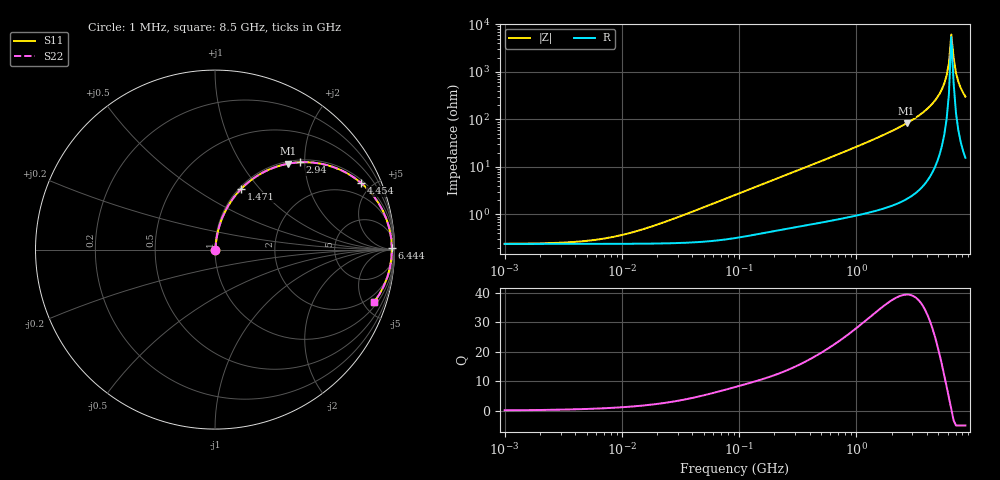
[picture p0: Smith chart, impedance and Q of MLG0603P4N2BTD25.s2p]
! S-Parameter Data Generated by TDK Corporation
! Copyright(C) 2025 TDK Corporation.
! All Rights Reserved.
! TDK P/N: MLG0603P4N2BTD25 (SMD / SMT Inductor (Coil))
! Property: L=4.2nH at 500MHz
! Size(LxWxT): 0.6x0.3x0.3mm
! Model Type: s2p (Touchstone File Format Version 1.0)
! Frequency: DC=Yes Start=1MHz Stop=8500MHz 198points Log-sweep
! Model Generated on Feb. 6, 2025
! Terms and conditions regarding TDK Simulation Models:
! 1)This simulation model is being provided solely for informational
!  purposes. Please refer to the specifications of the products in
!  terms of detailed characteristics of such products.
! 2)In no event shall TDK Corporation of any of its subsidiaries be
!  liable for any loss or damage arising, directly or indirectly,
!  from any information contained in this simulation model, including,
!  but not limited to loss or damages arising from any inaccuracies,
!  omissions or errors in connection with such information.
! 3)Any and all copyrights on this simulation model are owned by
!  TDK Corporation.  Duplication or redistribution of this simulation
!  model without prior written permission from TDK Corporation
!  is prohibited.
! 4)This simulation model is subject to any modification or change
!  without any prior notice.
! 5)Neither TDK Corporation nor any of its subsidiaries shall make any
!  warranty, express or implied, including but not limited to the
!  correctness, implied warranties of merchantability and fitness for
!  a particular purpose with respect to this simulation models.
! 6)The use of this simulation model shall be deemed to have consented
!  to the terms and conditions hereof.
! Port Assignments:
!  1 ---@@@--- 2
! Applicable Conditions:
!  Temperature = 25 degC
!  DC Bias Current = 0 A
!  Small Signal Operation
# Hz S MA R 50
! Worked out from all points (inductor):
!   197 points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, 1 MHz to 8.5 GHz, reference 50 ohm
!   read as one part in series: L = 4.45 nH near 27.76 MHz
!   highest Q = 39.3 at 2.681 GHz (marker M1), where L = 4.91 nH
!   self-resonance near 6.444 GHz
!   S11 on the Smith chart (normalised r, x): 1 MHz: 1.00, +0.00; 1.471 GHz: 1.02, +0.80; 2.94 GHz: 1.05, +1.89; 4.454 GHz: 1.15, +4.30; 6.444 GHz: open; 8.5 GHz: 1.31, -6.01
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1000000  0.002411 6.6  0.9976 -0.0  0.9976 -0.0  0.002411 6.6
4587603  0.002718 28.1  0.9976 -0.1  0.9976 -0.1  0.002718 28.1
9601846  0.003604 48.0  0.9976 -0.2  0.9976 -0.2  0.003604 48.0
2.10461e7  0.006367 67.1  0.9975 -0.3  0.9975 -0.3  0.006367 67.1
9.219544e7  0.02554 81.4  0.9965 -1.5  0.9965 -1.5  0.02554 81.4
4.229561e8  0.1107 80.5  0.9877 -6.3  0.9877 -6.3  0.1107 80.5
8.852465e8  0.2262 74.8  0.9655 -13.1  0.9655 -13.1  0.2262 74.8
1.470933e9  0.3673 66.7  0.9192 -21.5  0.9192 -21.5  0.3673 66.7
1.940355e9  0.4749 60.1  0.8673 -28.3  0.8673 -28.3  0.4749 60.1
2.680511e9  0.6299 49.5  0.7608 -39.0  0.7608 -39.0  0.6299 49.5
2.939772e9  0.679 45.8  0.717 -42.7  0.717 -42.7  0.679 45.8
3.703002e9  0.8038 34.9  0.5726 -53.5  0.5726 -53.5  0.8038 34.9
4.453958e9  0.8946 24.6  0.4158 -63.4  0.4158 -63.4  0.8946 24.6
5.357206e9  0.9605 12.9  0.2235 -73.5  0.2235 -73.5  0.9605 12.9
5.87536e9  0.9789 6.7  0.1178 -76.4  0.1178 -76.4  0.9789 6.7
6.152938e9  0.9838 3.6  0.06399 -73.6  0.06399 -73.6  0.9838 3.6
6.44363e9  0.9856 0.4  0.01614 -26.9  0.01614 -26.9  0.9856 0.4
6.748056e9  0.9844 -2.7  0.04978 70.3  0.04978 70.3  0.9844 -2.7
7.066863e9  0.9801 -5.9  0.1034 76.0  0.1034 76.0  0.9801 -5.9
7.400733e9  0.9727 -9.0  0.157 75.5  0.157 75.5  0.9727 -9.0
7.750377e9  0.9626 -12.1  0.2097 73.7  0.2097 73.7  0.9626 -12.1
8.5e9  0.9345 -18.1  0.3107 68.9  0.3107 68.9  0.9345 -18.1
